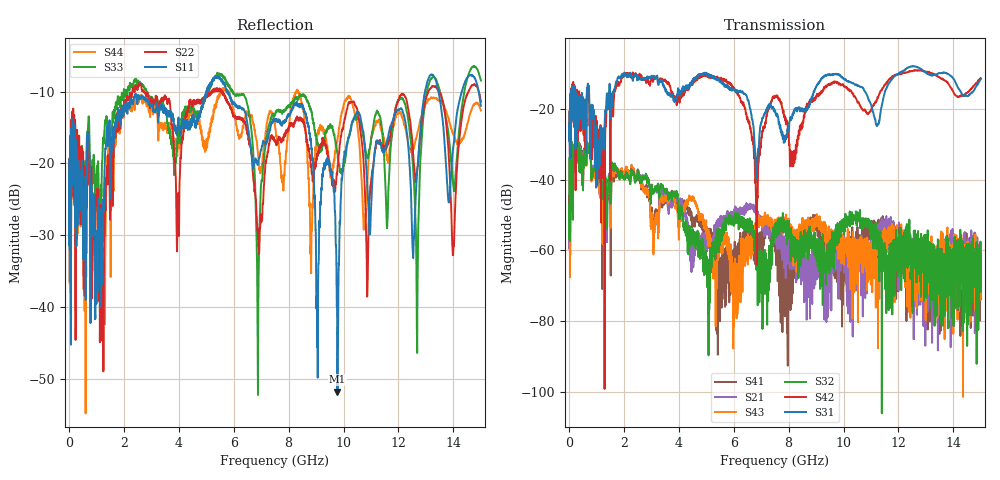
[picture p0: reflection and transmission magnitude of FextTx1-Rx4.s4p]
! FILE: N:\QM 2007\Prüfprotokolle\Highspeed\Konfektionierte Ltg\L45593-D106\D30\8216\0002\Fext\FextTx1-Rx4.s4p
# MHz S RI R 50.00
! FREQ  S11  S12  S13  S14
!  S21  S22  S23  S24
!  S31  S32  S33  S34
!  S41  S42  S43  S44
!  REAL  IMAG  REAL  IMAG  REAL  IMAG  REAL  IMAG
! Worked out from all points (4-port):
!   2999 points, 10 MHz to 15 GHz, reference 50 ohm
!   strongest paths, dB at 10 MHz, 3.755 GHz, 7.505 GHz, 11.26 GHz, 15 GHz:
!     S31: -24.5, -15.9, -20.7, -24.3, -11.5
!     S42: -25.2, -15.4, -16.9, -16.9, -11.5
!     S32: -47.3, -46.0, -53.3, -56.6, -71.7
!     S43: -44.7, -44.3, -54.2, -87.7, -61.1
!     S21: -50.1, -47.7, -57.8, -53.5, -70.6
!     S41: -52.4, -43.2, -59.8, -53.5, -67.2
!   lowest |S11| = -51.8 dB at 9.78 GHz (marker M1), VSWR 1.01, Z = 50 - j0.256 ohm
!   |S11| at or under -10 dB: start of sweep to 5.006 GHz; 5.781 GHz to 12.96 GHz (7.184 GHz wide, 76.6 % of centre); 13.46 GHz to 14.3 GHz (845.4 MHz wide, 6.09 % of centre)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
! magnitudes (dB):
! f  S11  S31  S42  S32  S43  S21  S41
! 10 MHz  -19.4  -24.5  -25.2  -47.3  -44.7  -50.1  -52.4
! 5.665 GHz  -8.7  -13.8  -11.9  -52.8  -56.7  -51.8  -67.3
! 6.84 GHz  -19.7  -36.8  -64.1  -60.4  -51.9  -49.5  -60.2
! 9.78 GHz  -51.8  -10.4  -12.7  -57.2  -56.5  -62.9  -63.7
! 10.46 GHz  -13.1  -13.1  -17.2  -52.4  -62.9  -60.4  -58.5
! 12.68 GHz  -21.4  -8.2  -9.2  -61.5  -62.4  -78.3  -73.6
! 15 GHz  -12.0  -11.5  -11.5  -71.7  -61.1  -70.6  -67.2
